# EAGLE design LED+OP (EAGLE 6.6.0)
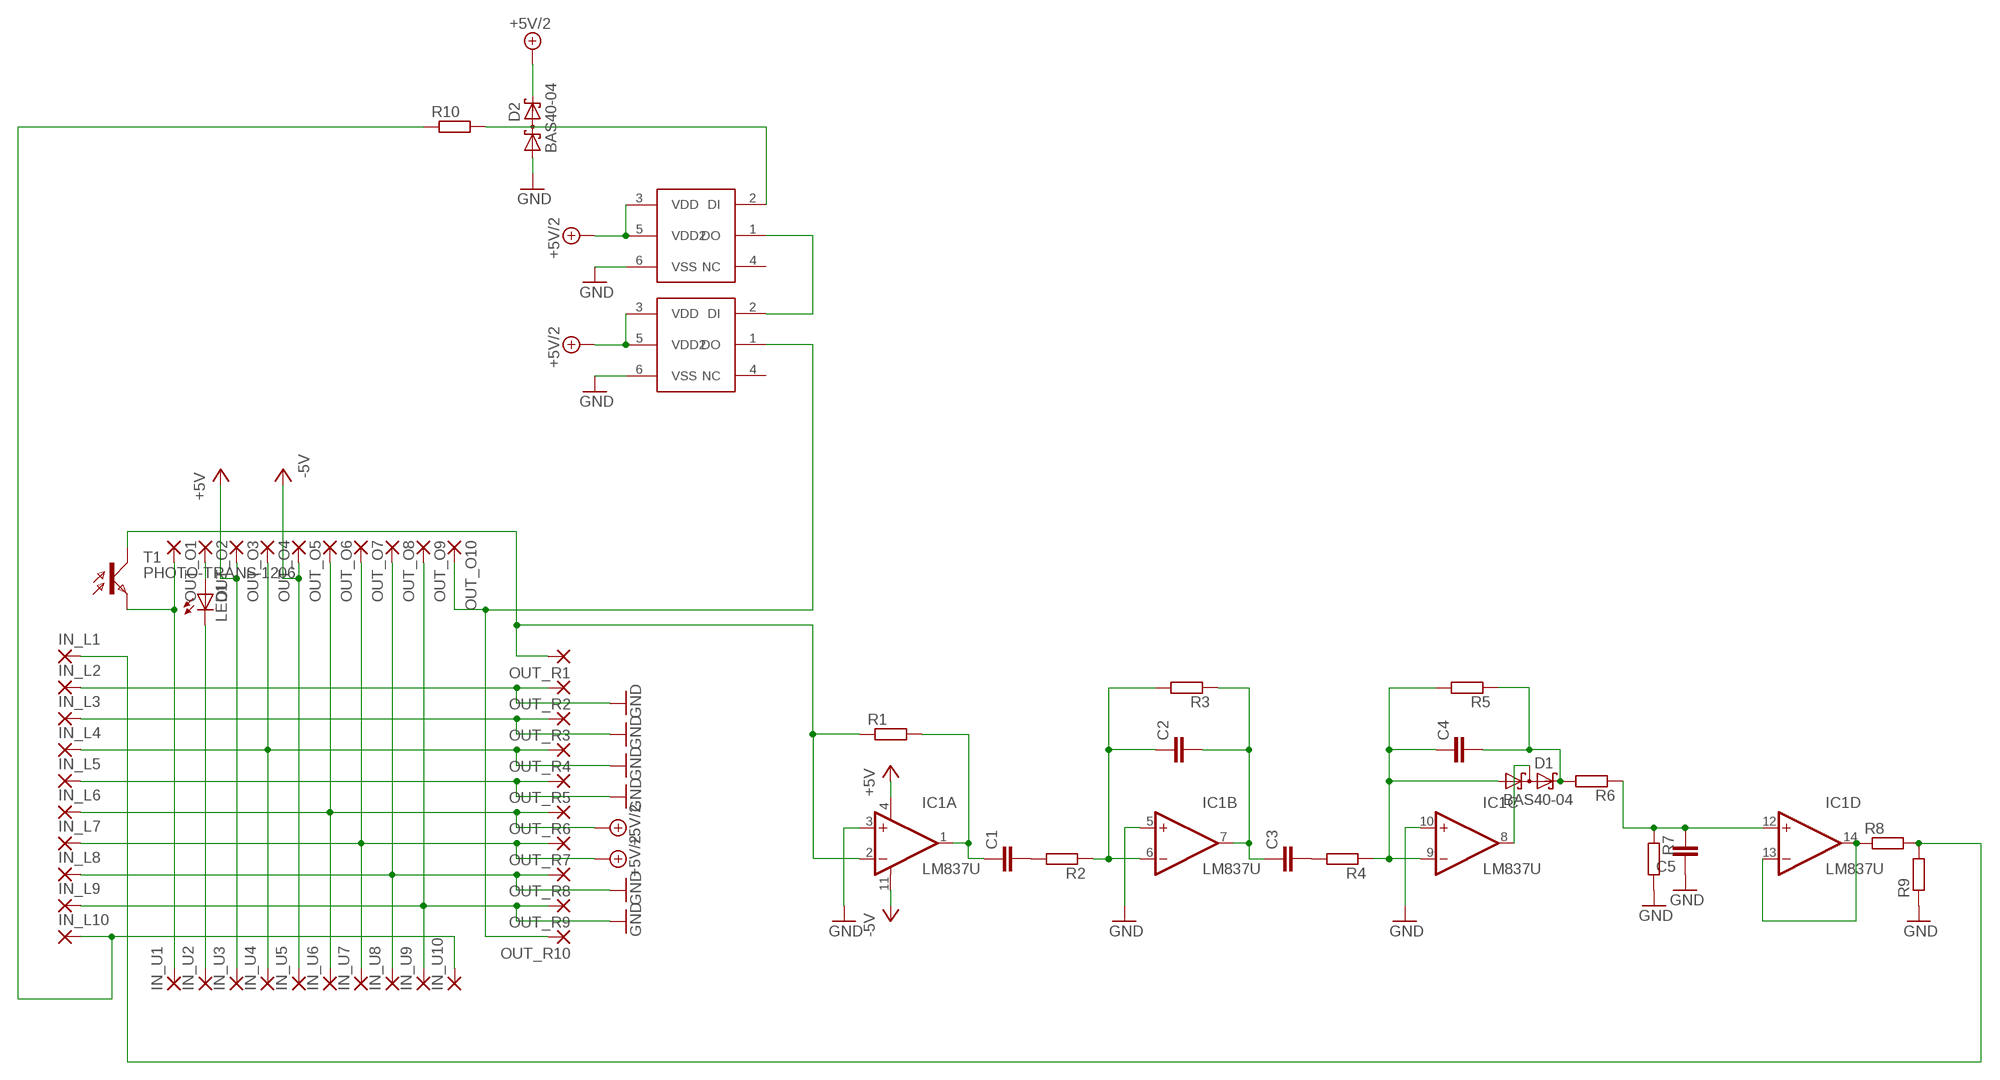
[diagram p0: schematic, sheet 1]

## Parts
C1  C-EUC1206  [C1206]
C2  C-EUC1206  [C1206]
C3  C-EUC1206  [C1206]
C4  C-EUC1206  [C1206]
C5  C-EUC1206  [C1206]
D1  BAS40-04  [SOT23]
D2  BAS40-04  [SOT23]
IC1  LM837U  [SO14]
IN_L  SMD2  [SMD1,27-2,54]
IN_U  SMD2  [SMD1,27-2,54]
LED1  LED3MM  [LED3MM]
OUT_O  SMD2  [SMD1,27-2,54]
OUT_R  SMD2  [SMD1,27-2,54]
R1  R-EU_M1206  [M1206]
R2  R-EU_M1206  [M1206]
R3  R-EU_M1206  [M1206]
R4  R-EU_M1206  [M1206]
R5  R-EU_M1206  [M1206]
R6  R-EU_M1206  [M1206]
R7  R-EU_M1206  [M1206]
R8  R-EU_M1206  [M1206]
R9  R-EU_M1206  [M1206]
R10  R-EU_M1206  [M1206]
T1  PHOTO-TRANS-1206  [1206]
U$1  LED_SMD5050  [CLN6A]
U$2  LED_SMD5050  [CLN6A]

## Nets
+5V: IC1.4(A:V+) IN_U.3 OUT_O.3
+5V/2: D2.2(C2) IN_L.6 IN_L.7 IN_U.6 IN_U.7 OUT_O.6 OUT_O.7 OUT_R.6 OUT_R.7 U$1.3(VDD) U$1.5(VDD2) U$2.3(VDD) U$2.5(VDD2)
-5V: IC1.11(A:V-) IN_U.5 OUT_O.5
GND: C5.1 D2.1(A1) IC1.3(A:+IN) IC1.5(B:+IN) IC1.10(C:+IN) IN_L.2 IN_L.3 IN_L.4 IN_L.5 IN_L.8 IN_L.9 IN_U.4 IN_U.8 IN_U.9 OUT_O.4 OUT_O.8 OUT_O.9 OUT_R.2 OUT_R.3 OUT_R.4 OUT_R.5 OUT_R.8 OUT_R.9 R7.2 R9.1 U$1.6(VSS) U$2.6(VSS)
N$1: IC1.2(A:-IN) OUT_R.1 R1.1 T1.A(C)
N$2: C1.1 IC1.1(A:OUT) R1.2
N$3: C1.2 R2.2
N$4: IN_U.1 OUT_O.1 T1.C(E)
N$5: D1.3(C1A2) IC1.8(C:OUT)
N$6: U$1.1(DO) U$2.2(DI)
N$7: D2.3(C1A2) R10.2 U$1.2(DI)
N$8: IC1.13(D:-IN) IC1.14(D:OUT) R8.1
N$9: C2.1 IC1.6(B:-IN) R2.1 R3.2
N$10: C2.2 C3.1 IC1.7(B:OUT) R3.1
N$11: C4.2 D1.2(C2) R5.1 R6.2
N$13: LED1.A OUT_O.2
N$14: C3.2 R4.2
N$15: C4.1 D1.1(A1) IC1.9(C:-IN) R4.1 R5.2
N$16: OUT_O.10 OUT_R.10 U$2.1(DO)
N$17: IN_L.10 IN_U.10 R10.1
N$18: IN_L.1 R8.2 R9.2
N$19: C5.2 IC1.12(D:+IN) R6.1 R7.1
N$25: IN_U.2 LED1.K(C)
Unconnected: U$1.4(NC) U$2.4(NC)

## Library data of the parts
C1-C5 = resistor:C-EU: CAPACITOR, European symbol
D1 D2 = diode:BAS40-04: Silicon Schottky Diodes General-purpose diode for high-speed switching
IC1 = #mylib:LM837: Operational Amplifiers; OC_FARNELL: unknown; OC_NEWARK: unknown
IN_L IN_U OUT_O OUT_R = #mylib:SMD2: SMD PAD
LED1 = led:LED: LED
R1-R10 = resistor:R-EU_: RESISTOR, European symbol
T1 = #mylib:PHOTO-TRANS-1206: PHOTO TRANSISTOR
U$1 U$2 = #mylib:LED_SMD5050

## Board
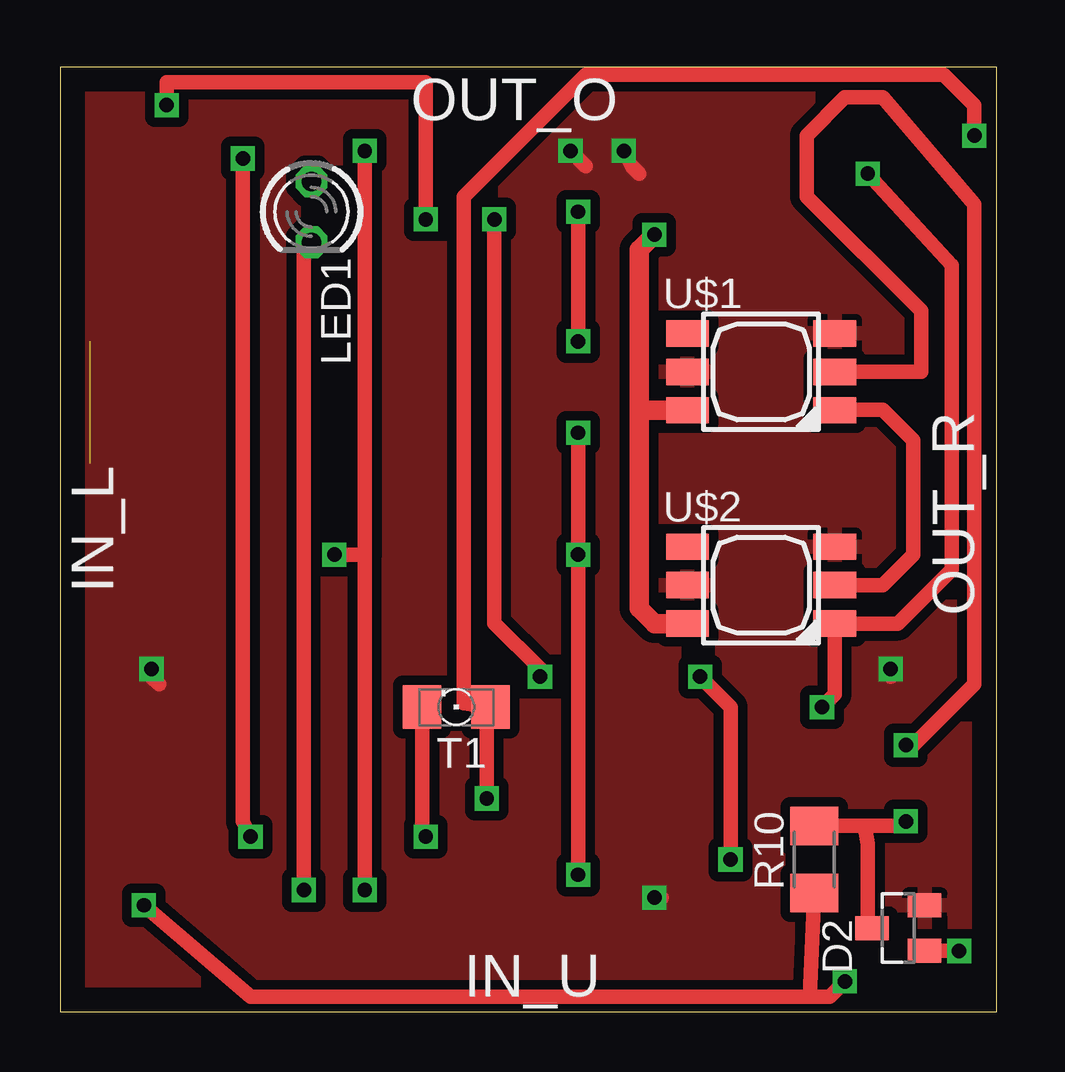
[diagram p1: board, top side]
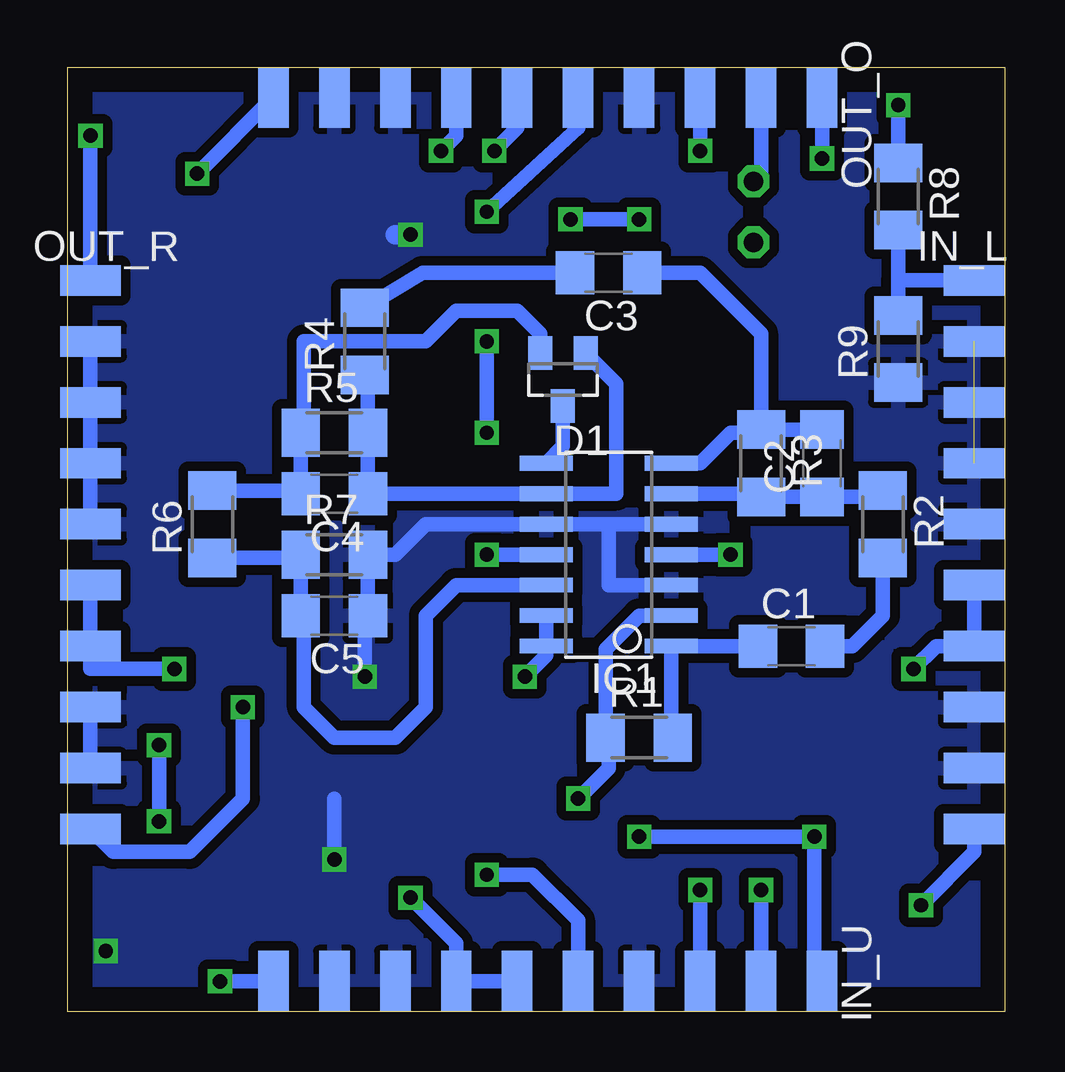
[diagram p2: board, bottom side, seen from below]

Size 39.04 x 39.36 mm. Coordinates in mm from the lower left corner, seen from the top.
Outline: 0,0 39.04,0 39.04,39.36 0,39.36 0,0
Copper layers (1*16): Top 0.035mm / dielectric 1.5mm / Bottom 0.035mm
Design rules "default": minimum track width 10mil, minimum drill 0.6mm, track to track 8mil, track to pad 8mil, pad to pad 8mil, via to via 8mil, smd to smd 8mil, copper to edge 40mil, drill to drill 8mil, minimum pad ring 10mil, minimum via ring 8mil, stop-mask expansion 4mil, vias tented up to drill 0mil, thermal gap 10mil

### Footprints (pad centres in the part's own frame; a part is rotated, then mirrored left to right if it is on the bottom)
C1206 = smd 1.6 x 1.8: 1 -1.4,0; 2 1.4,0
SOT23 = smd 1 x 1.4: 1 -0.95,-1.1; 2 0.95,-1.1; 3 0,1.1
SO14 = smd 0.61 x 2.21: 1 -3.81,-2.603; 2 -2.54,-2.603; 3 -1.27,-2.603; 4 0,-2.603; 5 1.27,-2.603; 6 2.54,-2.603; 7 3.81,-2.603; 8 3.81,2.603; 9 2.54,2.603; 10 1.27,2.603; 11 0,2.603; 12 -1.27,2.603; 13 -2.54,2.603; 14 -3.81,2.603
SMD1,27-2,54 = smd 1.27 x 2.54: 1 0,0; 2 2.54,0; 3 5.08,0; 4 7.62,0; 5 10.16,0; 6 12.7,0; 7 15.24,0; 8 17.78,0; 9 20.32,0; 10 22.86,0
LED3MM = drill 0.813 octagon: A -1.27,0; K 1.27,0
M1206 = smd 1.6 x 2: 1 -1.4,0; 2 1.4,0
1206 = smd 1.6 x 1.803: A -1.422,0; C 1.422,0
CLN6A = smd 1.778 x 1.1: 1 3.071,-1.6; 2 3.071,0; 3 3.071,1.6; 4 -3.071,1.6; 5 -3.071,0; 6 -3.071,-1.6

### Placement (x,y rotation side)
C1  8.89,15.24 0 bottom
C2  7.62,22.86 90 bottom
C3  16.51,30.8 180 bottom
C4  27.94,21.59 180 bottom
C5  27.94,16.51 180 bottom
D1  18.41,26.35 180 bottom
D2  34.92,3.49 90 top
IC1  16.51,19.05 90 bottom
IN_L  1.27,30.48 270 bottom
IN_U  7.62,1.27 180 bottom
LED1  10.48,33.34 270 top
OUT_O  7.62,38.1 180 bottom
OUT_R  38.1,30.48 270 bottom
R1  15.24,11.43 0 bottom
R2  5.08,20.32 270 bottom
R3  10.16,22.86 270 bottom
R4  26.67,27.94 90 bottom
R5  27.94,24.13 0 bottom
R6  33.02,20.32 90 bottom
R7  27.94,19.05 0 bottom
R8  4.45,33.97 270 bottom
R9  4.45,27.62 90 bottom
R10  31.43,6.35 90 top
T1  16.51,12.7 180 top
U$1  29.21,26.67 0 top
U$2  29.21,17.78 0 top

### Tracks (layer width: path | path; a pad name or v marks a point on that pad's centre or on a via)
+5V  (via drill 0.6)
  Top 0.61: v12.7,5.08 12.7,19.05 | 12.7,19.05 v11.43,19.05 | v12.7,35.88 12.7,19.05
  Bottom 0.61: IN_U.3 v12.7,5.08 | v11.43,19.05 IC1.4 | OUT_O.3 v12.7,35.88
+5V/2  (via drill 0.6)
  Top 0.61: v21.27,35.88 21.91,35.24 | v23.5,35.88 23.81,35.24 24.13,34.92 | v3.81,14.29 3.81,13.97 4.13,13.65 | v24.77,4.76 25.08,4.76 | v34.61,14.29 34.61,13.97
  Bottom 0.61: OUT_O.6 20.32,36.83 v21.27,35.88 | OUT_O.7 22.86,36.51 v23.5,35.88 | IN_L.6 IN_L.7 2.86,15.24 v3.81,14.29 | IN_U.6 IN_U.7 22.86,2.86 v24.77,4.76 | OUT_R.7 OUT_R.6 38.1,14.29 v34.61,14.29
  pour Top (isolate 0.406): 0,39.37 38.1,39.37 37.78,0.32 0,0
-5V  (via drill 0.6)
  Top 0.61: v21.59,5.71 v21.59,19.05 v21.59,24.13 | v21.59,33.34 v21.59,27.94
  Bottom 0.61: IC1.11 v21.59,19.05 | v21.59,27.94 v21.59,24.13 | v21.59,33.34 17.78,36.83 OUT_O.5 | v21.59,5.71 19.68,5.71 17.78,3.81 IN_U.5
GND  (via drill 0.6)  (2 unrouted)
  Top 0.61: v26.67,13.97 27.94,12.7 v27.94,6.35 | D2.1 v37.46,2.54 v37.47,2.54
  Top 0.813: U$2.6 24.78,16.18 24.13,16.83 24.13,25.08 | 24.13,25.08 24.13,31.75 v24.77,32.38 | U$1.6 24.14,25.07 24.13,25.08
  Bottom 0.61: 16.51,20.32 IC1.10 24.13,20.32 25.4,19.05 R7.2 C5.1 26.67,16.38 v26.67,13.97 | 16.51,20.32 IC1.5 | IC1.3 16.51,17.78 16.51,20.32 | 27.94,8.89 v27.94,6.35 | OUT_R.2 OUT_R.3 OUT_R.4 OUT_R.5 | OUT_R.8 OUT_R.9
  Bottom 0.813: v24.77,32.38 25.4,32.38
  pour Bottom (isolate 0.406): 0,39.37 38.1,39.37 38.1,0 0,0
N$1  (via drill 0.6)
  Top 0.61: v17.78,8.89 17.78,12.55 T1.A 16.83,12.87 16.83,33.97 21.91,39.05 36.83,39.05 38.1,37.78 v38.1,36.51
  Bottom 0.61: IC1.2 15.24,16.51 16.64,15.11 R1.1 16.51,11.43 16.51,10.16 v17.78,8.89 | OUT_R.1 v38.1,36.51
N$2
  Bottom 0.61: C1.1 IC1.1 13.91,11.5 R1.2
N$3
  Bottom 0.61: R2.2 5.08,16.51 6.35,15.24 C1.2
N$4  (via drill 0.6)
  Top 0.61: v7.62,35.56 7.62,7.94 v7.94,7.3 | T1.C 15.09,7.46 v15.24,7.3
  Bottom 0.61: OUT_O.1 v7.62,35.56 | IN_U.1 7.94,1.59 v7.94,7.3 v15.24,7.3
N$5
  Bottom 0.61: 19.05,22.92 IC1.8 18.41,23.56 D1.3
N$6
  Top 0.61: U$2.2 34.29,17.78 35.56,19.05 35.56,23.81 34.29,25.08 32.29,25.08 U$1.1
N$7  (via drill 0.6)
  Top 0.61: R10.2 33.52,7.75 | 33.52,7.75 33.66,6.99 33.66,3.66 D2.3 | 33.52,7.75 35.11,7.75 v35.24,7.94 | v35.24,11.11 35.56,11.11 38.1,13.65 38.1,33.66 34.29,38.1 32.7,38.1 31.11,36.51 31.11,33.97 35.88,29.21 35.88,26.67 U$1.2
  Bottom 0.61: v35.24,7.94 v35.24,11.11
N$8  (via drill 0.6)
  Top 0.61: v20,13.97 20,14.29 18.1,16.19 v18.1,33.02 | v15.24,33.02 15.24,38.73 4.45,38.73 v4.45,37.78
  Bottom 0.61: IC1.14 IC1.13 19.11,14.86 v20,13.97 | v18.1,33.02 v15.24,33.02 | R8.1 v4.45,37.78
N$9
  Bottom 0.61: IC1.6 10.29,21.59 R3.2 C2.1 5.34,21.46 R2.1
N$10
  Bottom 0.61: IC1.7 12.7,22.86 11.43,24.13 10.29,24.13 R3.1 | R3.1 C2.2 | C3.1 12.7,30.8 10.16,28.26 R3.1
N$11
  Bottom 0.61: R6.2 29.47,21.72 C4.2 R5.1 29.21,24.26 29.21,27.94 24.13,27.94 22.86,29.21 20.32,29.21 19.36,28.25 D1.2
N$13
  Bottom 0.61: OUT_O.2 10.16,34.92 LED1.A
N$14
  Bottom 0.61: R4.2 24.26,30.8 C3.2
N$15
  Bottom 0.61: R4.1 26.54,26.41 R5.2 C4.1 IC1.9 16.19,21.59 16.19,26.18 D1.1
N$16  (via drill 0.6)
  Top 0.61: v31.75,12.7 32.28,13.23 U$2.1 34.91,16.18 37.15,18.41 37.15,31.11 v33.66,34.92
  Bottom 0.61: v31.75,12.7 31.75,8.89 33.97,6.67 37.15,6.67 OUT_R.10 | v33.66,34.92 OUT_O.10
N$17  (via drill 0.6)
  Top 0.61: v3.49,4.45 7.94,0.64 31.25,0.64 | 31.25,0.64 R10.1 | 31.25,0.64 32.07,0.64 v32.7,1.27
  Bottom 0.61: IN_L.10 1.27,6.67 v3.49,4.45 | v32.7,1.27 IN_U.10
N$18
  Bottom 0.61: R8.2 4.45,30.48 | 4.45,30.48 R9.2 | IN_L.1 4.45,30.48
N$19
  Bottom 0.61: R7.1 C5.2 29.21,16.38 29.21,12.7 27.94,11.43 25.4,11.43 24.13,12.7 24.13,16.51 22.86,17.78 IC1.12 | R6.1 29.47,18.92 R7.1 | R7.1 29.21,19.05
N$25  (via drill 0.6)
  Top 0.61: v10.16,5.08 10.16,31.75 LED1.K
  Bottom 0.61: IN_U.2 v10.16,5.08

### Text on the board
tNames: OUT_O | IN_L | OUT_R | IN_U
